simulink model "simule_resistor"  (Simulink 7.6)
settings: Solver=ode15s  StartTime=0.0  StopTime=10.0  RelTol=1e-3
InitFcn:
  | R=5;
StartFcn:
  | clc
StopFcn:
  | close all
  | load  I_R_Simscape.mat
  | plot(x(1,:),x(2,:))
  | hold on
  | plot(x(1,:),x(3,:))
  | axis([0 0.14 -1.2 1.2])
  | grid
  | title('Courant dans R et tension d''entrée')
  | xlabel('Simulation d''une résistance')
libraries: fl_lib x9, nesl_utility x4

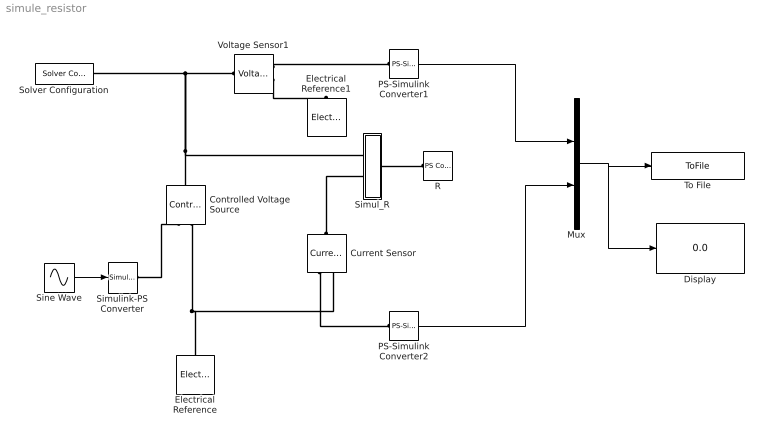
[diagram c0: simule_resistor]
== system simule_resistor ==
  Controlled Voltage Source : fl_lib/Electrical/Electrical Sources/Controlled Voltage Source  DialogController=NetworkEngine.DynNeDlgSource  SystemSampleTime=-1  i_Log=off  v_Log=off  LocalVarNames=|i|v  LocalVarDescs=|i|v  LocalVarLogging=[0 0]
  Current Sensor : fl_lib/Electrical/Electrical Sensors/Current Sensor  DialogController=NetworkEngine.DynNeDlgSource  SystemSampleTime=-1  i1_Log=off  v1_Log=off  LocalVarNames=|i1|v1  LocalVarDescs=|i1|v1  LocalVarLogging=[0 0]
  Display : Display
  Electrical Reference : fl_lib/Electrical/Electrical Elements/Electrical Reference  DialogController=NetworkEngine.DynNeDlgSource  SystemSampleTime=-1  i_Log=off  LocalVarNames=|i  LocalVarDescs=|i  LocalVarLogging=0
  Electrical Reference1 : fl_lib/Electrical/Electrical Elements/Electrical Reference  DialogController=NetworkEngine.DynNeDlgSource  SystemSampleTime=-1  i_Log=off  LocalVarNames=|i  LocalVarDescs=|i  LocalVarLogging=0
  Mux : Mux  Inputs=2
  PS-Simulink Converter1 : nesl_utility/PS-Simulink Converter  DialogController=NetworkEngine.DynNeUtilDlgSource  SystemSampleTime=-1  PhysicalDomain=network_engine_domain  LeftPortType=input  RightPortType=output  SubClassName=ps_output  Unit=1  AffineConversion=off
  PS-Simulink Converter2 : nesl_utility/PS-Simulink Converter  DialogController=NetworkEngine.DynNeUtilDlgSource  SystemSampleTime=-1  PhysicalDomain=network_engine_domain  LeftPortType=input  RightPortType=output  SubClassName=ps_output  Unit=1  AffineConversion=off
  R : fl_lib/Physical Signals/Sources/PS Constant  DialogController=NetworkEngine.DynNeDlgSource  SystemSampleTime=-1  constant=R  LocalVarLogging=[]
  Simul_R : Subsystem
  Simulink-PS Converter : nesl_utility/Simulink-PS Converter  DialogController=NetworkEngine.DynNeUtilDlgSource  SystemSampleTime=-1  PhysicalDomain=network_engine_domain  LeftPortType=input  RightPortType=output  SubClassName=ps_input  Unit=1  AffineConversion=off  InputFilterTimeConstant=.001  UdotUserProvided=0
  Sine Wave : Sin  Frequency=100  SampleTime=0
  Solver Configuration : nesl_utility/Solver Configuration  DialogController=NetworkEngine.DynNeUtilDlgSource  SystemSampleTime=-1  PhysicalDomain=network_engine_domain  LeftPortType=input  RightPortType=generic  SubClassName=solver  Accelerate=off  Profile=off  ResidualTolerance=1e-9  MaxNonlinIter=3  MaxModeIter=2  DoFixedCost=off  UseLocalSampling=off  DoDC=off  LinearAlgebra=Sparse  LocalSolverSampleTime=.001  LocalSolverChoice=NE_BACKWARD_EULER_ADVANCER  UseLocalSolver=off
  To File : ToFile  Filename=I_R_Simscape  MatrixName=x
  Voltage Sensor1 : fl_lib/Electrical/Electrical Sensors/Voltage Sensor  DialogController=NetworkEngine.DynNeDlgSource  SystemSampleTime=-1  i1_Log=off  v1_Log=off  LocalVarNames=|i1|v1  LocalVarDescs=|i1|v1  LocalVarLogging=[0 0]
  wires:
  Sine Wave/1 -> Simulink-PS Converter/1
  PS-Simulink Converter1/1 -> Mux/1
  PS-Simulink Converter2/1 -> Mux/2
  Mux/1 -> To File/1, Display/1
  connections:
  Controlled Voltage Source/RConn2 -- Electrical Reference/LConn1 -- Current Sensor/RConn2
  Simulink-PS Converter/RConn1 -- Controlled Voltage Source/RConn1
  Controlled Voltage Source/LConn1 -- Simul_R/LConn1 -- Voltage Sensor1/LConn1 -- Solver Configuration/RConn1
  Simul_R/RConn1 -- R/RConn1
  Voltage Sensor1/RConn1 -- PS-Simulink Converter1/LConn1
  Voltage Sensor1/RConn2 -- Electrical Reference1/LConn1
  Current Sensor/LConn1 -- Simul_R/LConn2
  Current Sensor/RConn1 -- PS-Simulink Converter2/LConn1

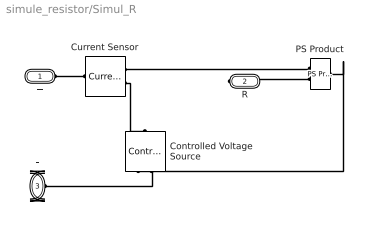
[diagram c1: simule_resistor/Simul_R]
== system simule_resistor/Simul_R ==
  Controlled Voltage Source : fl_lib/Electrical/Electrical Sources/Controlled Voltage Source  DialogController=NetworkEngine.DynNeDlgSource  SystemSampleTime=-1  i_Log=off  v_Log=off  LocalVarNames=|i|v  LocalVarDescs=|i|v  LocalVarLogging=[0 0]
  Current Sensor : fl_lib/Electrical/Electrical Sensors/Current Sensor  DialogController=NetworkEngine.DynNeDlgSource  SystemSampleTime=-1  i1_Log=off  v1_Log=off  LocalVarNames=|i1|v1  LocalVarDescs=|i1|v1  LocalVarLogging=[0 0]
  PS Product : fl_lib/Physical Signals/Functions/PS Product  DialogController=NetworkEngine.DynNeDlgSource  SystemSampleTime=-1  LocalVarLogging=[]
  + : PMIOPort  Port=1  Side=Left
  R : PMIOPort  Port=2  Side=Right
  - : PMIOPort  Port=3  Side=Left
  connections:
  Current Sensor/RConn2 -- Controlled Voltage Source/LConn1
  Controlled Voltage Source/RConn1 -- PS Product/RConn1
  Current Sensor/RConn1 -- PS Product/LConn1
  +/RConn1 -- Current Sensor/LConn1
  R/RConn1 -- PS Product/LConn2
  Controlled Voltage Source/RConn2 -- -/RConn1
